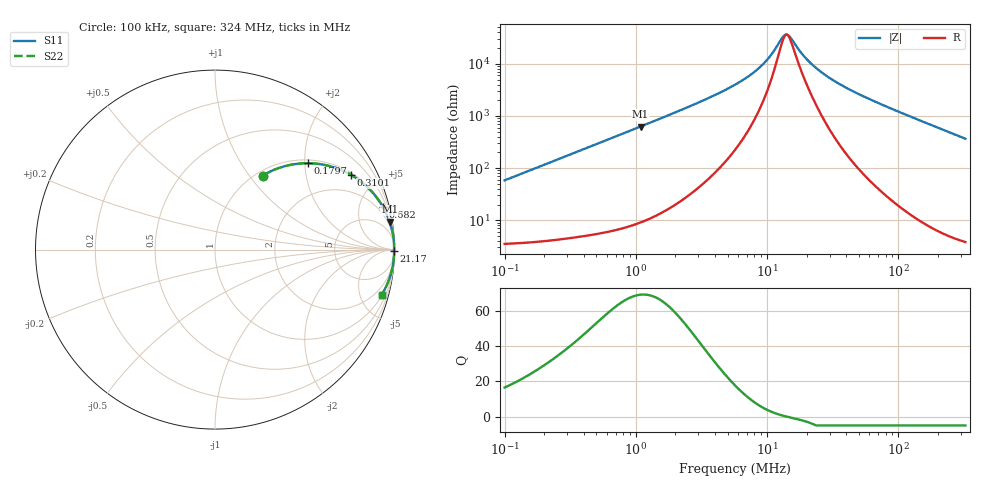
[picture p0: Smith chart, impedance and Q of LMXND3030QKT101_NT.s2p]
! LMXND3030QKT101_NT  S-PARAMETER MODEL  ( Standard Model )
! Model Generated by TAIYO YUDEN Corporation (https://www.yuden.co.jp/en/)
! Version 1.0
! TAIYO YUDEN Control No. 20250724
! Copyright(c) 2025 TAIYO YUDEN CO.,LTD. All Rights Reserved.
! Product Description (link to TY-COMPAS)
! https://ds.yuden.co.jp/TYCOMPAS/or/detail?pn=LMXND3030QKT101MNT&u=M
! Products Name : Inductors
! Characteristics :
!  Inductance : 100 [uH] , SRF(min) : 7.0 [MHz] , DC Resistance(max) : 2.88 [Ohm]
!  Rated Current : Saturation  230 [mA] , Temp Rise  320 [m A] (40 [degC])
!  Case Size : 3.0 x 3.0 / 0.118 x 0.118 [mm/inch] , Thickness : 1.5 / 0.059 [mm/inch]
!  (Conditions: Temperature = 25 [degC] , DC Bias Current = 0 [A])
! External Node Assignments :
!  1  o---GGG---o  2
! GND o---------o GND
! Frequency Range : 0.1MHz  -  324.04089MHz  [ 402 STEP ]
# MHz S RI R 50
! Freq[MHz].  S11 Real  S11 Imag  S21 Real  S21 Imag  S12 Real  S12 Imag  S22 Real  S22 Imag
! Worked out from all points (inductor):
!   401 points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, 100 kHz to 324 MHz, reference 50 ohm
!   read as one part in series: L = 92.2 uH near 104.1 kHz
!   highest Q = 69.3 at 1.085 MHz (marker M1), where L = 91.9 uH
!   self-resonance near 13.85 MHz
!   S11 on the Smith chart (normalised r, x): 100 kHz: 1.07, +1.16; 179.7 kHz: 1.08, +2.08; 310.1 kHz: 1.09, +3.58; 682 kHz: 1.13, +7.85; 21.17 MHz: open; 324 MHz: 1.08, -7.32
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0.1  0.2652 0.4123  0.7348 -0.4123  0.7348 -0.4123  0.2652 0.4123
0.179688  0.5187 0.4814  0.4813 -0.4814  0.4813 -0.4814  0.5187 0.4814
0.310087  0.7563 0.4169  0.2437 -0.4169  0.2437 -0.4169  0.7563 0.4169
0.38728  0.8274 0.3671  0.1726 -0.3671  0.1726 -0.3671  0.8274 0.3671
0.681973  0.9357 0.2373  0.0643 -0.2373  0.0643 -0.2373  0.9357 0.2373
1.085493  0.9731 0.1549  0.0269 -0.1549  0.0269 -0.1549  0.9731 0.1549
1.499861  0.9853 0.1129  0.0147 -0.1129  0.0147 -0.1129  0.9853 0.1129
3.365975  0.9964 0.0483  0.00361 -0.0483  0.00361 -0.0483  0.9964 0.0483
5.692459  0.998 0.025  0.00204 -0.025  0.00204 -0.025  0.998 0.025
7.402772  0.9981 0.0164  0.0019 -0.0164  0.0019 -0.0164  0.9981 0.0164
9.245617  0.9979 0.0101  0.00205 -0.0101  0.00205 -0.0101  0.9979 0.0101
10.86796  0.9977 0.006  0.00229 -0.006  0.00229 -0.006  0.9977 0.006
13.03576  0.9974 0.00176  0.0026 -0.00176  0.0026 -0.00176  0.9974 0.00176
13.85051  0.9973 0.000422  0.0027 -0.000422  0.0027 -0.000422  0.9973 0.000422
15.01661  0.9972 -0.00132  0.00279 0.00132  0.00279 0.00132  0.9972 -0.00132
18.01194  0.9972 -0.00524  0.00281 0.00524  0.00281 0.00524  0.9972 -0.00524
21.17251  0.9974 -0.00897  0.00264 0.00897  0.00264 0.00897  0.9974 -0.00897
22.04577  0.9974 -0.00997  0.00258 0.00997  0.00258 0.00997  0.9974 -0.00997
28.09593  0.9977 -0.0166  0.00229 0.0166  0.00229 0.0166  0.9977 -0.0166
37.2833  0.9977 -0.0259  0.00228 0.0259  0.00228 0.0259  0.9977 -0.0259
85.37896  0.9939 -0.0692  0.00608 0.0692  0.00608 0.0692  0.9939 -0.0692
324.0409  0.9283 -0.2529  0.0717 0.2529  0.0717 0.2529  0.9283 -0.2529
